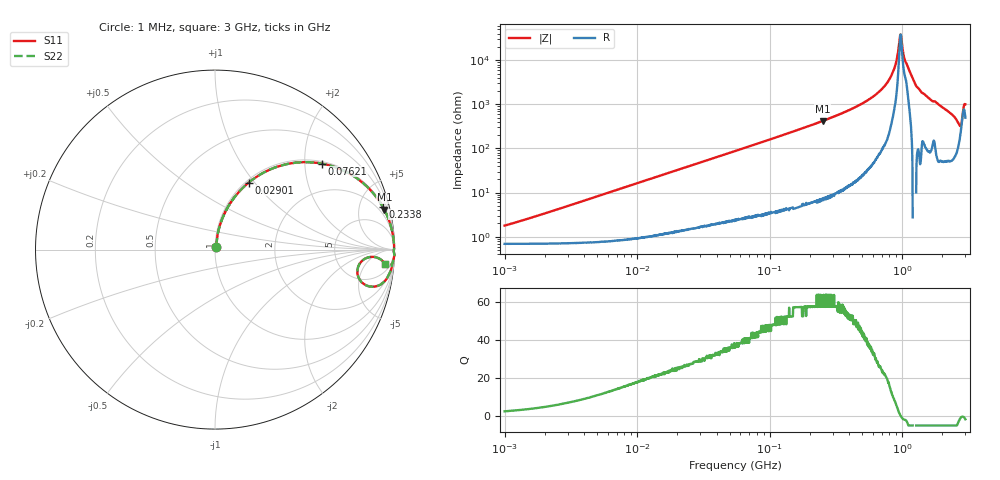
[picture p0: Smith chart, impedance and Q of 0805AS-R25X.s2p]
!s-Parameter Generated by FASTRON Sdn. Bhd.
!FASTRON P/N : 0805AS-R25X
!Keysight Technologies: E4991B_MY54100416_A.01.15
!Date: Mon Jun 15 12:53:26 2026
!Version  :Rev01  Mon Jun 15 12:53:26 2026
!Data & Calibration Information:
!Freq  S11  S21  S12  S22
!PortZ  Port1:50+j0  Port2:50+j0
!When reading reference impedance value at option line is always used.
! Remarks : This data is being provided solely for informational purposes.
# Hz S dB R 50
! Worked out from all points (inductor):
!   1601 points, 1 MHz to 3 GHz, reference 50 ohm
!   read as one part in series: L = 262 nH near 1.259 MHz
!   highest Q = 63.5 at 252 MHz (marker M1), where L = 267 nH
!   self-resonance near 973.1 MHz
!   S11 on the Smith chart (normalised r, x): 1 MHz: 1.01, +0.03; 29.01 MHz: 1.03, +0.93; 76.21 MHz: 1.06, +2.43; 233.8 MHz: 1.13, +7.75; 3 GHz: 11, -17
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1000000  -35.00 66.4  -0.06 -0.9  -0.06 -0.9  -35.00 66.4
3804036  -24.10 79.8  -0.08 -3.5  -0.08 -3.5  -24.10 79.8
1.447069e7  -12.90 74.3  -0.32 -13.1  -0.32 -13.1  -12.90 74.3
2.90111e7  -7.59 63.4  -0.97 -24.6  -0.97 -24.6  -7.59 63.4
5.504702e7  -3.73 47.8  -2.60 -40.6  -2.60 -40.6  -3.73 47.8
7.620648e7  -2.35 38.9  -4.03 -49.7  -4.03 -49.7  -2.35 38.9
2.083556e8  -0.40 16.2  -11.10 -72.8  -11.10 -72.8  -0.40 16.2
2.3377e8  -0.32 14.4  -12.10 -74.6  -12.10 -74.6  -0.32 14.4
2.519921e8  -0.27 13.3  -12.80 -75.7  -12.80 -75.7  -0.27 13.3
5.337858e8  -0.05 4.8  -21.50 -83.7  -21.50 -83.7  -0.05 4.8
7.925923e8  -0.02 1.6  -31.00 -85.0  -31.00 -85.0  -0.02 1.6
8.760197e8  -0.02 0.8  -36.60 -82.1  -36.60 -82.1  -0.02 0.8
9.490412e8  -0.02 0.2  -47.70 -58.0  -47.70 -58.0  -0.02 0.2
9.730857e8  -0.02 0.0  -51.70 -3.0  -51.70 -3.0  -0.02 0.0
1.059487e9  -0.04 -0.6  -39.30 64.4  -39.30 64.4  -0.04 -0.6
1.147801e9  -0.02 -1.1  -34.50 83.0  -34.50 83.0  -0.02 -1.1
1.268618e9  -0.00 -2.1  -28.60 88.1  -28.60 88.1  -0.00 -2.1
1.402151e9  -0.04 -3.1  -25.40 83.5  -25.40 83.5  -0.04 -3.1
2.335937e9  -0.23 -9.1  -16.00 76.1  -16.00 76.1  -0.23 -9.1
2.673854e9  -1.03 -13.4  -12.20 56.6  -12.20 56.6  -1.03 -13.4
2.769173e9  -1.89 -9.6  -12.20 33.0  -12.20 33.0  -1.89 -9.6
3e9  -0.45 -4.7  -20.50 55.5  -20.50 55.5  -0.45 -4.7
